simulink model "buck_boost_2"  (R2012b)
settings: Solver=ode45  StartTime=0.0  StopTime=10.0  RelTol=1e-3
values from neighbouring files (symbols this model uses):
  C = 100e-6    (= 0.0001)    [boost_up1.m]    (also in buck_boost1.m = 0.0002; buck_boost2.m = 0.0002; buck_down1.m; buck_down2.m)
  f0 = 0.2e5    (= 20000)    [boost_up1.m]    (also in buck_boost1.m; buck_boost2.m; buck_down1.m; buck_down2.m)
  L = 0.001    [boost_up1.m]    (also in buck_boost1.m; buck_boost2.m; buck_down1.m; buck_down2.m)
  R = 5    [boost_up1.m]    (also in buck_boost1.m; buck_boost2.m; buck_down1.m = 2*Rmax,; buck_down2.m = 0.1*Rmax,)
  T = 1/f0    (= 5e-05)    [boost_up1.m]    (also in buck_boost1.m; buck_boost2.m; buck_down1.m; buck_down2.m)
  T1 = T-T2    (= 2.5e-05)    [buck_boost1.m]    (also in buck_boost2.m = 1e-05; sepic1.m = T-T2; sepic2.m = T-T2; unwucht_4.m = 500)
  Ui = 5    [boost_up1.m]    (also in buck_boost1.m; buck_boost2.m; buck_down1.m; buck_down2.m)

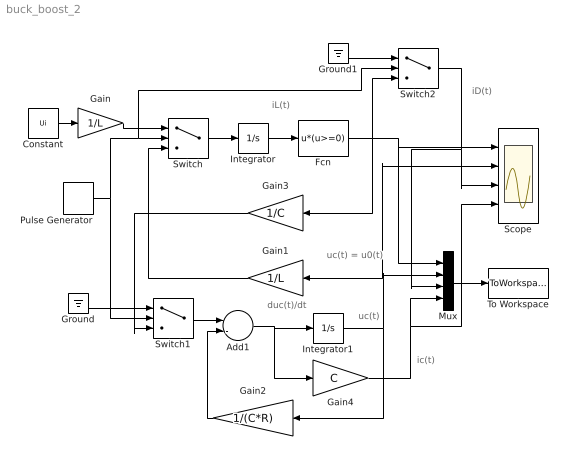
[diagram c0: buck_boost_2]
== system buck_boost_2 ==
  note: ic(t)
  note: uc(t)
  note: duc(t)/dt
  note: iD(t)
  note: uc(t) = u0(t)
  note: iL(t)
  Add1 : Sum  Inputs=--
  Constant : Constant  Value=Ui
  Fcn : Fcn  Expr=u*(u>=0)
  Gain : Gain  Gain=1/L
  Gain1 : Gain  Gain=1/L
  Gain2 : Gain  Gain=1/(C*R)
  Gain3 : Gain  Gain=1/C
  Gain4 : Gain  Gain=C
  Ground : Ground
  Ground1 : Ground
  Integrator : Integrator
  Integrator1 : Integrator
  Mux : Mux
  Pulse Generator : DiscretePulseGenerator  PulseType=Time based  Period=1/f0  PulseWidth=T1*100/T
  Scope : Scope  NumInputPorts=4
  Switch : Switch  Criteria=u2 > Threshold  Threshold=0.5  ZeroCross=off  SampleTime=0
  Switch1 : Switch  Criteria=u2 > Threshold  Threshold=0.5  ZeroCross=off  SampleTime=0
  Switch2 : Switch  Criteria=u2 > Threshold  Threshold=0.5  ZeroCross=off  SampleTime=0
  To Workspace : ToWorkspace  VariableName=y  SampleTime=-1  SaveFormat=Structure With Time
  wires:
  Constant/1 -> Gain/1
  Gain/1 -> Switch/1
  Integrator/1 -> Fcn/1
  Switch/1 -> Integrator/1
  Switch1/1 -> Add1/1
  Gain2/1 -> Add1/2
  Gain1/1 -> Switch/3
  Fcn/1 -> Switch2/3, Mux/1, Scope/1, Gain3/1
  Integrator1/1 -> Scope/2, Gain1/1, Mux/2, Gain2/1
  Mux/1 -> To Workspace/1
  Add1/1 -> Gain4/1, Integrator1/1
  Ground/1 -> Switch1/1
  Gain3/1 -> Switch1/3
  Ground1/1 -> Switch2/1
  Pulse Generator/1 -> Switch1/2, Switch2/2, Switch/2
  Switch2/1 -> Mux/3, Scope/3
  Gain4/1 -> Mux/4, Scope/4
